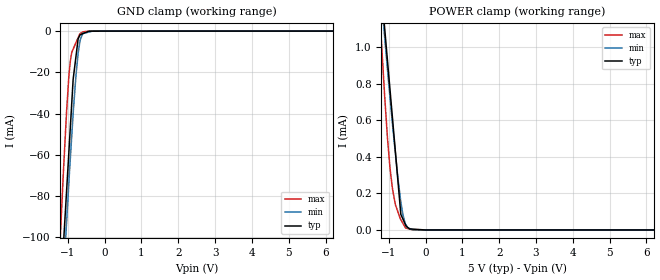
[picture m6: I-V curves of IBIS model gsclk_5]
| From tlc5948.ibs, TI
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|   gsclk_5 Model
[Model]   gsclk_5
Model_type   Input
Vinl = 1.5
Vinh = 3.5
|   typ   min   max
|   (nom PVT)   (fast PVT)   (slow PVT)
|C_comp from frequency sweep method (F=33MHz)
|Average
|C_comp   7.612e-13   7.432e-13   7.844e-13
|C_comp from LC tank measurement(L=1nH)
|Average
|Resonant Frequency(Hz)   6.940e+09   7.080e+09   6.760e+09
C_comp   5.264e-13   5.058e-13   5.549e-13
| Where nom  PVT is Nominal Process, 5V, 90C
|   Fast PVT is Strong Process,  5.5V, -40C
|   Slow PVT is Weak Process,   4.5V, 150C
[Model Spec]
|Subparameter   typ   min   max
Vinl   1.5   1.35   1.65
Vinh   3.5   3.15   3.85
[Voltage Range]   5   4.5   5.5
|Ambient Temperature   25   85   -40
|Junction Temperature
[Temperature Range]   90   150   -40
[Power Clamp Reference]   5   4.5   5.5
[GND Clamp Reference]   0   0   0
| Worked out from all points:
|   GND clamp passes 1 mA (typ) near -0.56 V on its own axis
|   POWER clamp passes 1 mA (typ) near -1.06 V on its own axis
[GND Clamp]
|   Voltage   I(typ)   I(min)   I(max)
-5V       -1.656A    -1.602A    -1.772A
-1.238V   -144.4mA   -159.7mA   -112.4mA
-1.14V    -110mA     -127.4mA   -75.89mA
-1.117V   -102.8mA   -119.6mA   -67.18mA
-1.062V   -86.29mA   -101.6mA   -48.73mA
-1.034V   -77.78mA   -92.95mA   -39.25mA
-962.5mV  -56.06mA   -70.76mA   -19.98mA
-907.5mV  -39.35mA   -54.84mA   -11.78mA
-855mV    -23.4mA    -39.98mA   -8.726mA
-720mV    -3.807mA   -10.81mA   -3.197mA
-594mV    -1.241mA   -1.204mA   -371.3uA
10V       0A         0A         0A
[POWER Clamp]
|   Voltage   I(typ)   I(min)   I(max)
-5V       12.85mA    11.04mA    15.23mA
-1.221V   1.415mA    1.312mA    1.114mA
-1.14V    1.176mA    1.126mA    838.7uA
-1.105V   1.096mA    1.047mA    722.3uA
-1.034V   929.8uA    882.4uA    506uA
-968mV    776.6uA    734.1uA    347.5uA
-891mV    598uA      567.1uA    218.4uA
-814mV    419.4uA    413uA      136.3uA
-670mV    85.3uA     153.6uA    55.91uA
-539mV    26.81uA    30.67uA    10.8uA
-229.5mV  3.135uA    95.48nA    29.91nA
10V       0A         0A         0A
